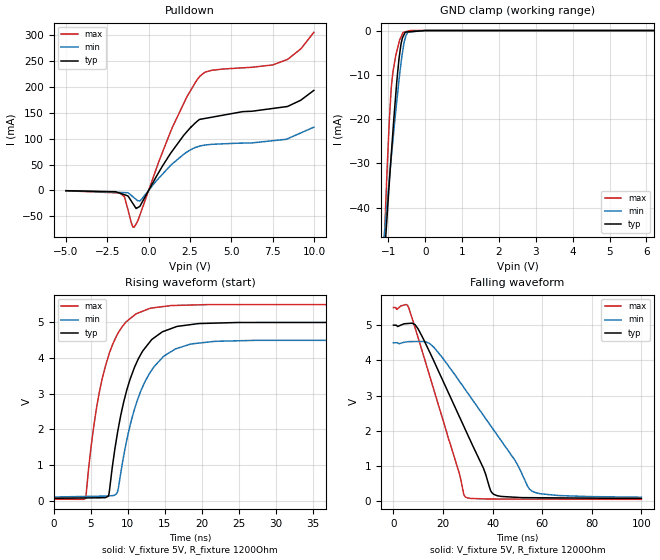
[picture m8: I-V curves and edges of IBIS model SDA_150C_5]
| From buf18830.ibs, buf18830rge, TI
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[Model] SDA_150C_5
|Signals SDA(15)
Model_type   I/O_open_drain
Polarity   Non-Inverting
Enable   Active-Low
Vinl = 1.5
Vinh = 3.5
Vmeas = 2.5
Vref = 2.5
Cref = 0pF
Rref = 10000
| Rpullup to DVDD = 1k
|   typ   min   max
|   (Nom PVT)   (Slow PVT)   (Fast PVT)
|  Output Low   9.72928E-13   8.09245E-13   1.16434E-12
|C_comp
|   Output High
C_comp   1.07172E-12   9.37736E-13   1.22484E-12
| Where   Nom PVT is  Nominal Process, 5.0V, 57C
|   Fast PVT is Strong Process, 5.5V, -40C
|   Slow PVT is Weak Process, 4.5V, 125C
[Model Spec]   |5V model
Vinl   1.5   1.35   1.65
Vinh   3.5   3.15   3.85
|Vinl = 0.3 X DVDD
|Vinh = 0.7 X DVDD
[Voltage Range]   5   4.5   5.5
|Operating Temperature   27   85   -40
[Temperature Range]   92   150   -40
[Pullup Reference]   5   4.5   5.5
[Pulldown Reference]   0   0   0
[Power Clamp Reference]   5   4.5   5.5
[GND Clamp Reference]   0   0   0
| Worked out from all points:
|   slope of the pulldown table from 0 to 0.75 V, typ, clamps not added: 17.7 ohm
|   GND clamp passes 1 mA (typ) near -0.58 V on its own axis
|   falling waveform, V_fixture 5V, R_fixture 1200Ohm: 20-80 % time 19.4ns typ, 25.9ns min, 14.1ns max; typ from 5 V to 0.073 V
|   rising waveform, V_fixture 5V, R_fixture 1200Ohm: 20-80 % time 3.53ns typ, 3.88ns min, 3.17ns max; typ from 0.073 V to 5 V
[Pulldown]
|   Voltage   I(typ)   I(min)   I(max)
-5V       -644uA     -466uA     -664.8uA
-1.737V   -5.429mA   -3.973mA   -5.099mA
-1.46V    -8.446mA   -4.271mA   -12.59mA
-1.058V   -20.2mA    -9.479mA   -61.76mA
-876.6mV  -29.19mA   -14.32mA   -71.06mA
-531.9mV  -30.95mA   -20.32mA   -48.11mA
1.458V    77.59mA    52.12mA    123.7mA
2.316V    113.8mA    74.25mA    181.4mA
3.101V    137.5mA    85.83mA    221.1mA
3.809V    141.6mA    89.16mA    232.4mA
8.392V    162.5mA    99.86mA    253.6mA
9.985V    193.6mA    122.4mA    306mA
[GND Clamp]
|   Voltage   I(typ)   I(min)   I(max)
-5V       -576.6mA   -428.7mA   -1.001A
-1.127V   -53.4mA    -47.56mA   -50.73mA
-1.045V   -43.07mA   -39.98mA   -33.25mA
-976.1mV  -34.47mA   -33.67mA   -20.46mA
-909mV    -26.45mA   -27.51mA   -11.74mA
-804.9mV  -14.93mA   -18.54mA   -5.868mA
-710.8mV  -6.281mA   -11.04mA   -2.645mA
-649.9mV  -2.734mA   -6.835mA   -1.306mA
-597.1mV  -1.274mA   -3.835mA   -414.4uA
-471.6mV  -312.4uA   -350uA     -138.5uA
1.655mV   0A         0A         0A
9.985V    0A         0A         0A
[POWER Clamp]
|   SCR cell for ESD function. Effects occurr above VDD x 2
|   Voltage   I(typ)   I(min)   I(max)
-5V       0A         0A         0A
0V        0A         0A         0A
10V       0A         0A         0A
[Ramp]
R_load = 1200
|   typ   min   max
dV/dt_r   2.95618/3.52308e-009   2.63502/3.86759e-009   3.27074/3.17132e-009
dV/dt_f   2.95618/1.93701e-008   2.63502/2.59459e-008   3.27074/1.40555e-008
[Falling Waveform]
V_fixture = 5V
V_fixture_min = 4.5V
V_fixture_max = 5.5V
R_fixture = 1200Ohm
C_fixture = 0F
|   Time   V(typ)   V(min)   V(max)
0s        5V         4.5V       5.5V
6.171ns   5.049V     4.533V     5.493V
9.909ns   4.899V     4.535V     4.655V
15.37ns   4.123V     4.433V     3.38V
29.03ns   2.026V     3.164V     116.6mV
36.34ns   927.1mV    2.43V      61.74mV
39.6ns    247.8mV    2.104V     57.58mV
49.11ns   107.5mV    1.148V     56.2mV
55.85ns   95.24mV    284.2mV    55.21mV
100ns     73.03mV    108.3mV    48.77mV
[Rising Waveform]
V_fixture = 5V
V_fixture_min = 4.5V
V_fixture_max = 5.5V
R_fixture = 1200Ohm
C_fixture = 0F
|   Time   V(typ)   V(min)   V(max)
0s        73.03mV    108.3mV    48.77mV
4.32ns    82.96mV    124.7mV    73.06mV
5.783ns   86.33mV    130.2mV    2.585V
7.361ns   129mV      137.1mV    4.026V
8.619ns   1.902V     247.6mV    4.669V
9.885ns   3.114V     1.714V     5.031V
12.92ns   4.435V     3.564V     5.387V
16.48ns   4.873V     4.26V      5.475V
21.73ns   4.979V     4.469V     5.497V
100ns     5V         4.5V       5.5V
